FUNCTION_BLOCK Example24a_autoloading_sending //1 flyway 1 xbot (actual physical) - autoloading delete,create,activate,holdforzoneready,unload
VAR_INPUT
	Execute : BOOL;
END_VAR
VAR_OUTPUT
	Done : BOOL;
END_VAR
VAR_IN_OUT
	PM_Controller : PMControllerType;	// the planar motor controller to use
END_VAR
VAR
	PMC_AutoLoadingZone_Delete1 : PMC_AutoLoadingZone_Delete;
	xbotID_array78 : ARRAY[0..77] OF USINT;
	posx_array78 : ARRAY[0..77] OF REAL;
	posy_array78 : ARRAY[0..77] OF REAL;
	PMC_AutoDrivingMotion1 : PMC_AutoDrivingMotion;
	PMC_AutoLoadingZone_Create1 : PMC_AutoLoadingZone_Create;
	PMC_AutoLoadingZone_Activate1 : PMC_AutoLoadingZone_Activate;
	PMC_AutoLoadingZone_HoldForZoneReady1 : PMC_AutoLoadingZone_HoldForZoneReady;
	PMC_XYMotion1 : PMC_XYMotion;
	PMC_AutoLoadingZone_UnloadXbot1 : PMC_AutoLoadingZone_UnloadXbot;
END_VAR

//1 flyway 1 xbot (actual physical) - autoloading delete,create,activate,holdforzoneready,unload

//delete any existing zone
PMC_AutoLoadingZone_Delete1(Execute := Execute,ZoneID := 0,PM_Controller := PM_Controller);

//move xbot to starting positions
xbotID_array78[0] := 1;
posx_array78[0] := 0.06;
posy_array78[0] := 0.06;
PMC_AutoDrivingMotion1(Execute := PMC_AutoLoadingZone_Delete1.Done,nXbots := 1,RoutingType := 0,ZoneID := 0,XbotID := xbotID_array78,PosX := posx_array78,PosY := posy_array78,PM_Controller := PM_Controller);

//create an autoloading unloading zone on the top left edge (75,240) of the flyway 
PMC_AutoLoadingZone_Create1(Execute := PMC_AutoDrivingMotion1.Done,ZoneID := 1,ZoneMode := 0,UnloadingMode := 0,
					ZoneCenterX := 0.075,ZoneCenterY := 0.24,ZoneLength := 0.12,ZoneWidth := 0.15,MaxXbotSizeX := 0.12,MaxXbotSizeY := 0.12,
					MaxVel := 1,MaxAcc := 10,MaxHeight := 0,PM_Controller := PM_Controller);
					
//activate the unloading zone
PMC_AutoLoadingZone_Activate1(Execute := PMC_AutoLoadingZone_Create1.Done,ZoneID := 1,PM_Controller := PM_Controller);

//hold until the unloading zone is ready to receive a new xbot
PMC_AutoLoadingZone_HoldForZoneReady1(Execute := PMC_AutoLoadingZone_Activate1.Done,ZoneID := 1,PM_Controller := PM_Controller);

//move the xbot into the unloading zone
PMC_XYMotion1(Execute := PMC_AutoLoadingZone_HoldForZoneReady1.Done,cmdLB := 1,XbotID := 1,Mode := 0,Type_ := 0,PosX := PMC_AutoLoadingZone_HoldForZoneReady1.ZoneX,PosY := PMC_AutoLoadingZone_HoldForZoneReady1.ZoneY,EndVel := 0,MaxVel := 1,MaxAcc := 10,PM_Controller := PM_Controller);

//unload the xbot
PMC_AutoLoadingZone_UnloadXbot1(Execute := PMC_XYMotion1.Done,ZoneID := 1,XbotID := 1,PM_Controller := PM_Controller);

Done := PMC_AutoLoadingZone_UnloadXbot1.Done;

END_FUNCTION_BLOCK
